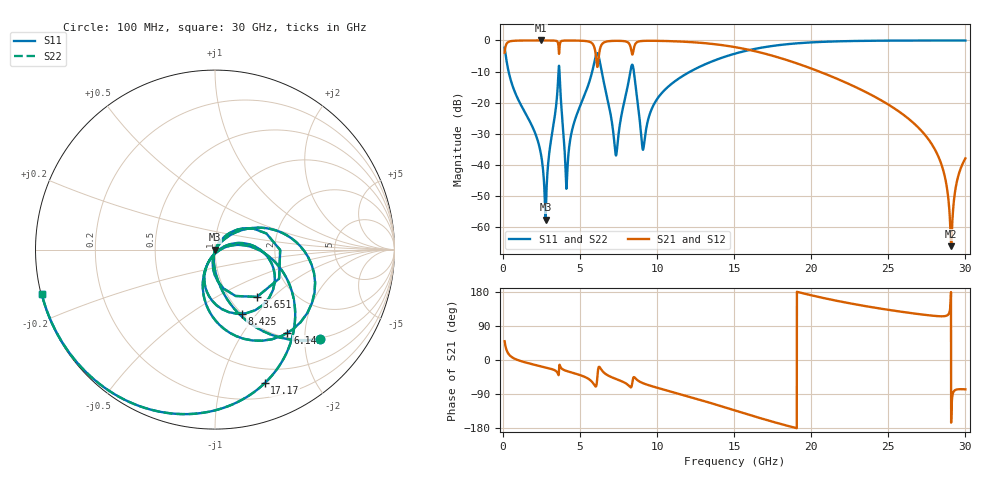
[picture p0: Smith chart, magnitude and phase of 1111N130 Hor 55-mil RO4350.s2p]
# GHz S MA R 50
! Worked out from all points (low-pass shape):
!   3201 points, 100 MHz to 30 GHz, reference 50 ohm
!   highest |S21| = -0.01 dB at 2.455 GHz (marker M1); lowest = -66.0 dB at 29.07 GHz (marker M2)
!   |S21| within 3 dB of the highest: 120.4 MHz to 3.61 GHz (3.49 GHz wide, 187 % of centre); 8.468 GHz to 15.95 GHz (7.478 GHz wide, 61.3 % of centre)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
!   lowest |S11| = -57.6 dB at 2.754 GHz (marker M3), VSWR 1.00, Z = 50.1 - j0.0421 ohm
!   |S11| at or under -10 dB: 357.8 MHz to 3.599 GHz (3.242 GHz wide, 164 % of centre); 3.66 GHz to 5.785 GHz (2.124 GHz wide, 45 % of centre); 8.485 GHz to 12.15 GHz (3.661 GHz wide, 35.5 % of centre)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
!   |S22| runs from -57.6 to 0.0 dB; largest |S21 - S12| = 0
!   S11 on the Smith chart (normalised r, x): 100 MHz: 0.97, -2.37; 3.651 GHz: 1.33, -0.80; 6.145 GHz: 1.09, -1.62; 8.425 GHz: 1.00, -0.84; 17.17 GHz: 0.34, -1.38; 30 GHz: 0.00, -0.13
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0.1  0.769 -40.4  0.6389 49.6  0.6389 49.6  0.769 -40.4
0.5485  0.2097 -81.7  0.9772 8.2  0.9772 8.2  0.2097 -81.7
2.454625  0.01513 -102.5  0.9985 -16.5  0.9985 -16.5  0.01513 -102.5
2.753625  0.001324 -18.5  0.9984 -19.5  0.9984 -19.5  0.001324 -18.5
3.650625  0.3522 -48.5  0.6885 -14.3  0.6885 -14.3  0.3522 -48.5
4.127156  0.004634 0.4  0.9955 -29.1  0.9955 -29.1  0.004634 0.4
5.089563  0.1005 45.3  0.9881 -41.2  0.9881 -41.2  0.1005 45.3
5.809031  0.3344 19.9  0.8816 -59.4  0.8816 -59.4  0.3344 19.9
6.145406  0.6153 -49.1  0.3946 -32.0  0.3946 -32.0  0.6153 -49.1
6.463094  0.2615 -104.0  0.8954 -29.9  0.8954 -29.9  0.2615 -104.0
7.322719  0.01425 -51.4  0.9849 -50.0  0.9849 -50.0  0.01425 -51.4
8.425281  0.3872 -67.5  0.6224 -50.5  0.6224 -50.5  0.3872 -67.5
9.079344  0.01758 -50.4  0.9817 -61.2  0.9817 -61.2  0.01758 -50.4
10.06978  0.1217 12.4  0.9838 -74.0  0.9838 -74.0  0.1217 12.4
15.05  0.6136 -43.8  0.7807 -133.2  0.7807 -133.2  0.6136 -43.8
17.17103  0.7947 -69.7  0.5966 -159.1  0.5966 -159.1  0.7947 -69.7
20.03956  0.9311 -100.1  0.3512 170.4  0.3512 170.4  0.9311 -100.1
25.01978  0.9921 -138.4  0.09286 132.3  0.09286 132.3  0.9921 -138.4
28.04716  0.9965 -155.8  0.01731 116.2  0.01731 116.2  0.9965 -155.8
28.66384  0.9966 -159.0  0.006555 115.8  0.006555 115.8  0.9966 -159.0
29.07497  0.9967 -161.1  0.0004997 -165.3  0.0004997 -165.3  0.9967 -161.1
30  0.9966 -165.6  0.01281 -77.4  0.01281 -77.4  0.9966 -165.6
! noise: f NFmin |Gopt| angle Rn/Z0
0.1  0.0009007  0.8  2.47  0.000933
3.417  0.02358  0.7459  23.87  0.01787
6.743  0.05912  0.8002  46.49  0.0519
10.06  0.03707  0.5942  65.98  0.01212
13.39  0.04148  0.554  80.92  0.01021
16.7  0.05943  0.6282  95.75  0.01434
20.03  0.09778  0.7461  112.6  0.02499
23.35  0.1963  0.8651  130.9  0.05535
26.67  0.6235  0.9557  148.9  0.2295
30  2.211  0.9869  165.5  0.6431
